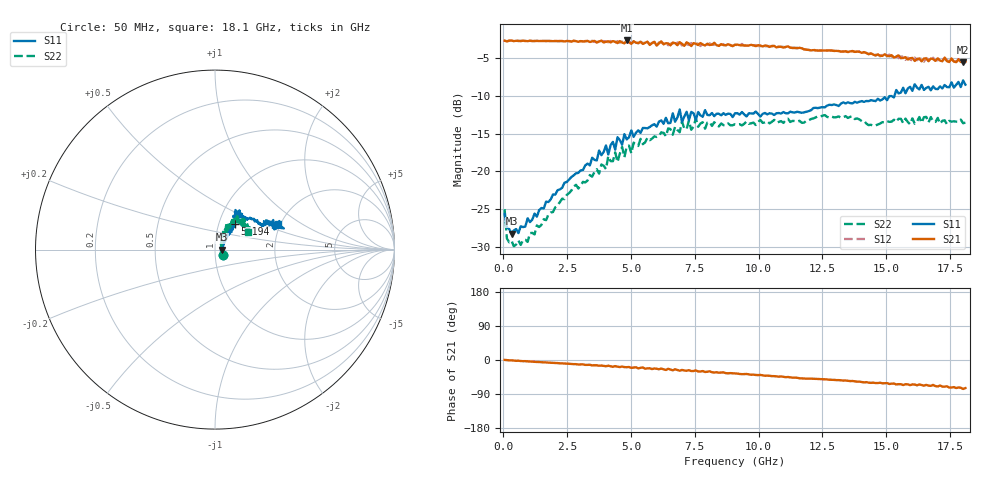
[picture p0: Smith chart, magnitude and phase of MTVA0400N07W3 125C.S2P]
! Network Analyzer HP8720D.06.14 Serial No. US36140669
!  8 Jul 2005  07:41:35
! Frequency  S11  S21  S12  S22
# HZ  S  DB R 50
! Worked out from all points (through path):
!   201 points, 50 MHz to 18.1 GHz, reference 50 ohm
!   highest |S21| = -2.63 dB at 4.833 GHz (marker M1); lowest = -5.5 dB at 18.01 GHz (marker M2)
!   group delay of S21, straight-line fit = 11.5 ps
!   lowest |S11| = -28.3 dB at 320.8 MHz (marker M3), VSWR 1.08, Z = 54 + j0.0037 ohm
!   |S11| at or under -10 dB: start of sweep to 15.32 GHz
!   |S22| runs from -29.9 to -12.5 dB; largest |S21 - S12| = 0.042
!   S11 on the Smith chart (normalised r, x): 50 MHz: 1.09, -0.06; 5.194 GHz: 1.20, +0.35; 18.1 GHz: 1.93, +0.63
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5e7  -25.65 -32.3  -2.66 0.3  -2.66 0.4  -25.05 -33.9
1.4025e8  -27.45 -16.5  -2.76 -0.3  -2.73 -0.4  -28.93 -18.5
3.2075e8  -28.28 0.1  -2.64 -0.9  -2.68 -0.9  -29.21 -2.1
9.525e8  -26.24 22.5  -2.72 -3.7  -2.66 -3.7  -29.37 26.8
3.1185e9  -19.84 48.6  -2.76 -11.5  -2.79 -12.0  -21.41 60.0
4.47225e9  -15.48 49.7  -2.98 -17.6  -2.73 -16.8  -18.77 65.5
4.65275e9  -16.47 50.4  -2.90 -17.2  -2.78 -18.9  -16.76 65.0
4.743e9  -15.07 53.6  -3.01 -18.8  -2.88 -17.8  -18.13 61.7
4.83325e9  -15.77 58.8  -2.63 -19.0  -2.90 -19.4  -16.72 55.8
5.19425e9  -14.88 51.7  -2.93 -19.1  -2.76 -19.8  -16.47 65.0
6.09675e9  -13.40 54.8  -3.01 -24.5  -2.89 -24.2  -15.30 57.9
6.7285e9  -13.42 61.4  -2.99 -24.3  -3.31 -25.1  -14.09 53.4
6.909e9  -11.79 58.1  -2.86 -28.4  -2.92 -26.2  -14.81 54.0
6.99925e9  -13.44 58.2  -3.08 -26.2  -3.31 -28.4  -13.40 54.5
7.36025e9  -12.11 53.1  -3.37 -29.2  -2.98 -28.3  -14.49 58.0
7.54075e9  -13.17 55.7  -3.08 -27.4  -2.99 -30.8  -13.00 56.4
7.90175e9  -11.88 57.4  -3.29 -31.6  -3.11 -29.8  -14.35 52.7
9.075e9  -12.30 55.9  -3.21 -35.5  -3.17 -35.7  -13.75 47.3
1.21435e10  -11.60 42.2  -3.91 -49.4  -3.85 -49.5  -12.98 48.3
1.512175e10  -10.02 26.5  -4.73 -63.2  -4.50 -62.6  -13.44 41.1
1.800975e10  -7.93 17.2  -5.55 -76.5  -5.30 -76.1  -13.62 33.2
1.81e10  -8.50 22.0  -5.45 -74.2  -5.74 -74.4  -13.54 28.5
